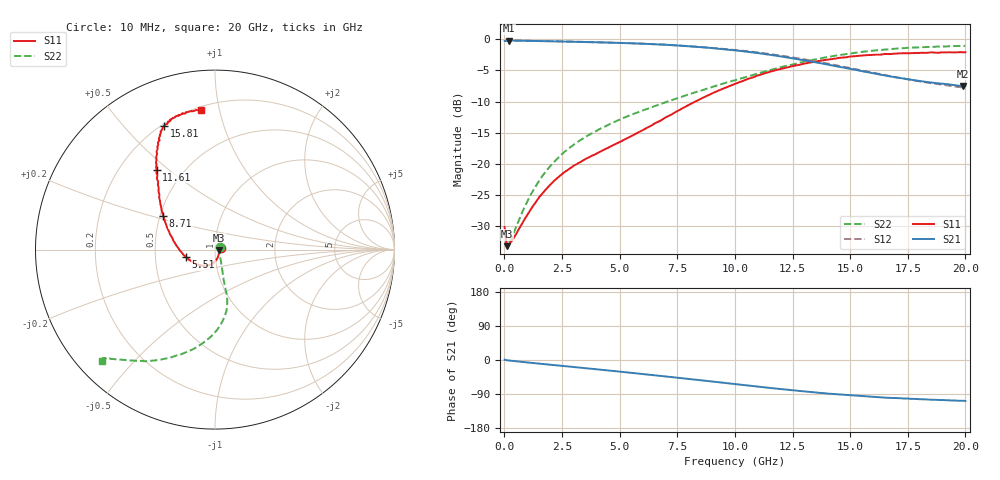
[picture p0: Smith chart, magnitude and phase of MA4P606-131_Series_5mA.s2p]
! AWR Design Environment (9226) Thu Aug 19 15:24:37 2021
! Document = '5mA'
! nPorts: 2, nXvals: 201
# GHz S DB R 50
!Freq DBS11 AngS11 DBS21 AngS21 DBS12 AngS12 DBS22 AngS22
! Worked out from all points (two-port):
!   201 points, 10 MHz to 20 GHz, reference 50 ohm
!   highest |S21| = -0.25 dB at 210 MHz (marker M1); lowest = -7.5 dB at 19.91 GHz (marker M2)
!   |S21| within 3 dB of the highest: start of sweep to 12.76 GHz
!   lowest |S11| = -33.2 dB at 110 MHz (marker M3), VSWR 1.04, Z = 52.2 - j0.365 ohm
!   |S11| at or under -10 dB: start of sweep to 8.287 GHz
!   |S22| runs from -33.2 to -1.1 dB; largest |S21 - S12| = 0.027
!   S11 on the Smith chart (normalised r, x): 10 MHz: 1.06, +0.01; 5.51 GHz: 0.72, -0.06; 8.71 GHz: 0.52, +0.22; 11.61 GHz: 0.36, +0.46; 15.81 GHz: 0.21, +0.65; 20 GHz: 0.22, +0.88
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0.01  -30.08 11.8  -0.31 0.8  -0.29 0.8  -30.55 25.1
0.11  -33.16 -9.2  -0.25 -0.8  -0.23 -0.7  -33.16 -10.9
0.21  -32.86 -16.7  -0.25 -1.4  -0.23 -1.4  -32.52 -18.6
1.11  -27.49 -66.4  -0.29 -7.2  -0.28 -7.0  -25.14 -57.7
1.61  -24.90 -81.6  -0.33 -10.2  -0.31 -10.0  -22.13 -64.2
2.01  -23.24 -91.7  -0.36 -12.6  -0.34 -12.3  -20.26 -67.8
2.51  -21.58 -103.2  -0.40 -15.6  -0.38 -15.2  -18.38 -70.7
3.41  -19.44 -122.2  -0.47 -21.0  -0.45 -20.4  -15.92 -73.3
4.41  -17.56 -143.1  -0.56 -27.0  -0.55 -26.4  -13.94 -74.7
5.51  -15.55 -165.5  -0.68 -33.7  -0.67 -32.9  -12.12 -75.1
6.71  -13.18 172.8  -0.86 -41.5  -0.85 -40.5  -10.50 -76.9
8.71  -9.24 146.7  -1.35 -54.7  -1.32 -53.5  -8.03 -83.6
10.01  -7.18 135.1  -1.80 -63.7  -1.74 -62.1  -6.60 -90.8
11.61  -5.16 126.1  -2.57 -74.3  -2.46 -72.7  -4.88 -102.7
13.41  -3.66 119.3  -3.67 -85.0  -3.52 -83.9  -3.32 -116.2
14.51  -3.02 115.7  -4.44 -90.9  -4.29 -89.9  -2.59 -123.5
15.81  -2.57 112.4  -5.35 -96.6  -5.25 -95.8  -1.93 -129.9
16.71  -2.41 109.5  -5.96 -99.9  -5.93 -99.0  -1.61 -132.7
18.01  -2.22 105.0  -6.71 -103.5  -6.78 -102.7  -1.32 -135.0
18.21  -2.21 105.2  -6.82 -103.6  -6.89 -103.4  -1.29 -135.5
19.91  -2.13 97.0  -7.52 -107.6  -7.75 -106.8  -1.09 -135.5
20  -2.11 95.9  -7.52 -108.1  -7.75 -107.0  -1.09 -135.6
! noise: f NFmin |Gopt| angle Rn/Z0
0.01  0  1  0  2e-20
2.21  0  1  0  2e-20
4.41  0  1  0  2e-20
6.61  0  1  0  2e-20
8.81  0  1  0  2e-20
11.11  0  1  0  2e-20
13.31  0  1  0  2e-20
15.51  0  1  0  2e-20
17.71  0  1  0  2e-20
20  0  1  0  2e-20
